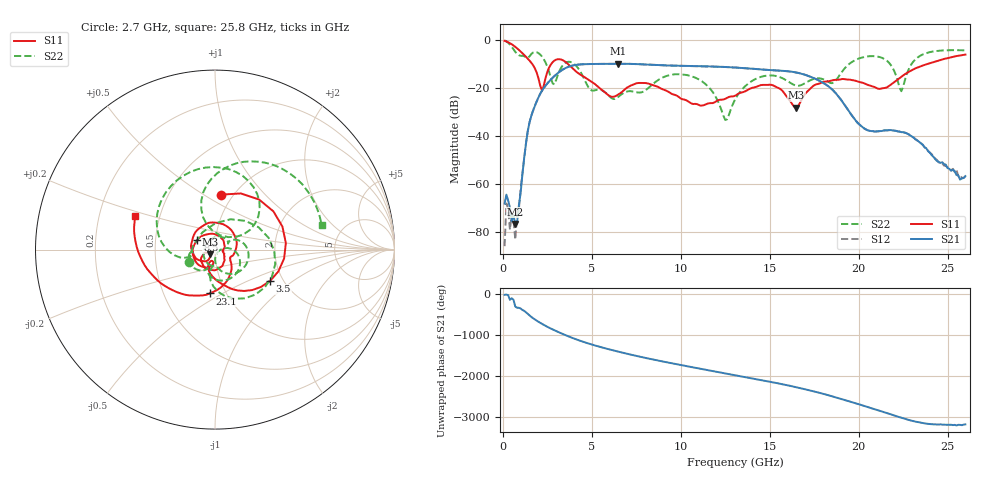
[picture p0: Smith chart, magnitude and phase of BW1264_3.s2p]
!Keysight Technologies,N5245B,MY57181159,A.13.60.06
!Date: Friday, December 18, 2020 23:52:05
!Correction: S11(Full 2 Port(1,2))
!S21(Full 2 Port(1,2))
!S12(Full 2 Port(1,2))
!S22(Full 2 Port(1,2))
!S2P File: Measurements: S11, S21, S12, S22:
# Hz S  dB  R 50
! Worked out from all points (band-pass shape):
!   260 points, 100 MHz to 26 GHz, reference 50 ohm
!   highest |S21| = -9.93 dB at 6.5 GHz (marker M1); lowest = -76.8 dB at 700 MHz (marker M2)
!   |S21| within 3 dB of the highest: 3.253 GHz to 15.82 GHz (12.56 GHz wide, 132 % of centre)
!   lowest |S11| = -28.3 dB at 16.5 GHz (marker M3), VSWR 1.08, Z = 47.3 - j2.58 ohm
!   |S11| at or under -10 dB: 1.649 GHz to 2.723 GHz (1.074 GHz wide, 49.1 % of centre); 3.656 GHz to 23.88 GHz (20.22 GHz wide, 147 % of centre)
!   |S22| runs from -33.4 to -0.2 dB; largest |S21 - S12| = 0.00051
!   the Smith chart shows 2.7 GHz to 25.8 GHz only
!   S11 on the Smith chart (normalised r, x): 2.7 GHz: 0.88, +0.60; 3.5 GHz: 1.71, -0.68; 8.5 GHz: 0.82, +0.09; 23.1 GHz: 0.84, -0.44; 25.8 GHz: 0.36, +0.18
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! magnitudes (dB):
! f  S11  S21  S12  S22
! 100 MHz  -0.4  -68.4  -86.1  -0.2
! 200 MHz  -0.6  -64.6  -68.3  -0.6
! 700 MHz  -2.9  -76.8  -83.4  -4.9
! 1.5 GHz  -8.6  -34.4  -34.4  -6.8
! 2.2 GHz  -21.1  -21.2  -21.2  -6.9
! 2.7 GHz  -10.2  -16.5  -16.5  -15.8
! 3.5 GHz  -9.0  -11.8  -11.8  -9.6
! 4.5 GHz  -15.1  -10.1  -10.1  -15.2
! 6.5 GHz  -22.7  -9.9  -9.9  -23.7
! 8.5 GHz  -19.0  -10.4  -10.4  -18.0
! 8.8 GHz  -19.9  -10.5  -10.5  -16.4
! 11.2 GHz  -27.4  -11.0  -11.0  -17.3
! 12.5 GHz  -24.6  -11.3  -11.3  -33.4
! 13.1 GHz  -23.1  -11.5  -11.5  -24.2
! 15.1 GHz  -18.7  -12.6  -12.6  -14.8
! 16.5 GHz  -28.3  -13.6  -13.6  -19.1
! 17.4 GHz  -19.5  -15.7  -15.7  -16.5
! 21.7 GHz  -19.2  -37.6  -37.7  -9.5
! 22.4 GHz  -15.3  -38.5  -38.3  -21.4
! 23.1 GHz  -12.2  -40.8  -40.8  -8.8
! 25.8 GHz  -6.3  -57.8  -57.6  -4.3
! 26 GHz  -6.1  -56.8  -57.0  -4.3
